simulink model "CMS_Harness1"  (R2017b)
settings: Solver=FixedStepDiscrete  StartTime=0.0  StopTime=2  FixedStep=0.01  RelTol=1e-3  EnableMultiTasking=on
undefined symbols (not defined in the file): sigbuilder_block
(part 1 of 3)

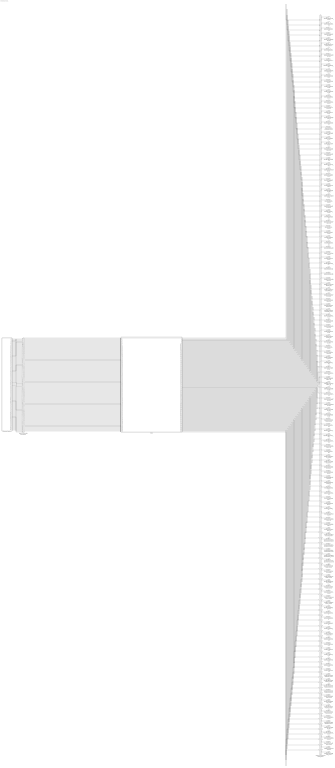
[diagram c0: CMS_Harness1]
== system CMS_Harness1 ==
  CMS : ModelReference  ModelNameDialog=CMS  SimulationMode=Normal  ModelReferenceVersion='M100C100'
  Harness Inputs : Subsystem  Tag=STV Subsys  LoadFcn=sigbuilder_block('load');  StartFcn=sigbuilder_block('start');  StopFcn=sigbuilder_block('stop');  ClipboardFcn=sigbuilder_block('clipboard');  mask(Sigbuilder block){tuvar=[0:10]}
      mask init:
      | if ~strcmp(get_param(bdroot(gcb),'SimulationStatus'),'stopped'),tuvar = sigbuilder_block('maskInit'); end
  Input Conversion Subsystem : Subsystem  Tag=__SLT_ICS__  Description=Signal spec. and routing
  Output Conversion Subsystem : Subsystem  Tag=__SLT_OCS__  Description=Signal spec. and routing
  GeCMS_HVConnSt_enum : Outport  OutDataTypeStr=uint8  PortDimensions=[1]
  GbCMS_NegCtlSt_flg : Outport  Port=2  OutDataTypeStr=boolean  PortDimensions=[1]
  GbCMS_PosCtlSt_flg : Outport  Port=3  OutDataTypeStr=boolean  PortDimensions=[1]
  GbCMS_ChrgPosCtlSt_flg : Outport  Port=4  OutDataTypeStr=boolean  PortDimensions=[1]
  GbCMS_ChrgNegCtlSt_flg : Outport  Port=5  OutDataTypeStr=boolean  PortDimensions=[1]
  GeCMS_RelStuckClosed_enum : Outport  Port=6  OutDataTypeStr=uint8  PortDimensions=[1]
  GcCMS_PackVolt_V : Outport  Port=7  OutDataTypeStr=fixdt('ufix16_Sp1')  PortDimensions=[1]
  GbCMS_PreChrgCtlSt_flg : Outport  Port=8  OutDataTypeStr=boolean  PortDimensions=[1]
  GcCMS_BattCurr_A : Outport  Port=9  OutDataTypeStr=fixdt('ufix16_Sp1_Bn700')  PortDimensions=[1]
  GbCMS_Kl15WkUp_flg : Outport  Port=10  OutDataTypeStr=boolean  PortDimensions=[1]
  GbCMS_ThmRunAway_flg : Outport  Port=11  OutDataTypeStr=boolean  PortDimensions=[1]
  GcCMS_CoolTempIn_C : Outport  Port=12  OutDataTypeStr=fixdt('ufix8_Bn40')  PortDimensions=[1]
  GcCMS_CoolTempOut_C : Outport  Port=13  OutDataTypeStr=fixdt('ufix8_Bn40')  PortDimensions=[1]
  GcCMS_CoolPwrReq_W : Outport  Port=14  OutDataTypeStr=fixdt('ufix16_Sp1')  PortDimensions=[1]
  GcCMS_HeatPwrReq_W : Outport  Port=15  OutDataTypeStr=fixdt('ufix16_Sp1')  PortDimensions=[1]
  GeCMS_CoolReq_enum : Outport  Port=16  OutDataTypeStr=uint8  PortDimensions=[1]
  GeCMS_HeatReq_enum : Outport  Port=17  OutDataTypeStr=uint8  PortDimensions=[1]
  GcCMS_PeakCurrDisCh_A : Outport  Port=18  OutDataTypeStr=fixdt('ufix16_Sp1')  PortDimensions=[1]
  GcCMS_PeakCurrCh_A : Outport  Port=19  OutDataTypeStr=fixdt('ufix16_Sp1_Bn1500')  PortDimensions=[1]
  GcCMS_PeakVoltDisCh_V : Outport  Port=20  OutDataTypeStr=uint16  PortDimensions=[1]
  GcCMS_PeakVoltCh_V : Outport  Port=21  OutDataTypeStr=uint16  PortDimensions=[1]
  GeCMS_Thm_propagat_enum : Outport  Port=22  OutDataTypeStr=uint8  PortDimensions=[1]
  GcCMS_ClntTgtTemp_C : Outport  Port=23  OutDataTypeStr=fixdt('ufix8_Bn40')  PortDimensions=[1]
  GcCMS_HtTgtTemp_C : Outport  Port=24  OutDataTypeStr=fixdt('ufix8_Bn40')  PortDimensions=[1]
  GcCMS_MaxCellVolt_V : Outport  Port=25  OutDataTypeStr=fixdt('ufix16_Sp001')  PortDimensions=[1]
  GcCMS_BusbarTempMax_C : Outport  Port=26  OutDataTypeStr=fixdt('ufix8_Bn40')  PortDimensions=[1]
  GcCMS_BusbarTempMin_C : Outport  Port=27  OutDataTypeStr=fixdt('ufix8_Bn40')  PortDimensions=[1]
  GcCMS_MinCellVolt_V : Outport  Port=28  OutDataTypeStr=fixdt('ufix16_Sp001')  PortDimensions=[1]
  GbCMS_ChrgCmd_flg : Outport  Port=29  OutDataTypeStr=boolean  PortDimensions=[1]
  GcCMS_ActPwrChrg_Kw : Outport  Port=30  OutDataTypeStr=fixdt('ufix16_Sp1')  PortDimensions=[1]
  GcCMS_MaxVoltChrg_V : Outport  Port=31  OutDataTypeStr=fixdt('ufix16_Sp1')  PortDimensions=[1]
  GcCMS_ReqVoltChrg_V : Outport  Port=32  OutDataTypeStr=fixdt('ufix16_Sp1')  PortDimensions=[1]
  GcCMS_ReqCurrChrg_A : Outport  Port=33  OutDataTypeStr=fixdt('ufix16_Sp1_Bn700')  PortDimensions=[1]
  GbCMS_ObcRdyReq_flg : Outport  Port=34  OutDataTypeStr=boolean  PortDimensions=[1]
  GbCMS_DischgCmd_flg : Outport  Port=35  OutDataTypeStr=boolean  PortDimensions=[1]
  GeCMS_BmsSt_enum : Outport  Port=36  OutDataTypeStr=uint8  PortDimensions=[1]
  GeCMS_BmsSelfChk_enum : Outport  Port=37  OutDataTypeStr=uint8  PortDimensions=[1]
  GeCMS_IsoFault_enum : Outport  Port=38  OutDataTypeStr=uint8  PortDimensions=[1]
  GcCMS_SocDspl_pct : Outport  Port=39  OutDataTypeStr=uint8  PortDimensions=[1]
  GbCMS_HvilOpenFault_flg : Outport  Port=40  OutDataTypeStr=boolean  PortDimensions=[1]
  GeCMS_FltLvl_enum : Outport  Port=41  OutDataTypeStr=uint8  PortDimensions=[1]
  GeCMS_V2xMod_enum : Outport  Port=42  OutDataTypeStr=uint8  PortDimensions=[1]
  GcCMS_ChgSOCset_pct : Outport  Port=43  OutDataTypeStr=fixdt('ufix8_B80')  PortDimensions=[1]
  GcCMS_BattSoh_pct : Outport  Port=44  OutDataTypeStr=uint8  PortDimensions=[1]
  GcCMS_SOCA_pct : Outport  Port=45  OutDataTypeStr=uint8  PortDimensions=[1]
  GeCMS_IviDischg_enum : Outport  Port=46  OutDataTypeStr=uint8  PortDimensions=[1]
  GcCMS_PackCurLem_A : Outport  Port=47  OutDataTypeStr=fixdt('ufix16_Bn1023')  PortDimensions=[1]
  GcCMS_BattInVolt_V : Outport  Port=48  OutDataTypeStr=fixdt('ufix16_Sp1')  PortDimensions=[1]
  GbCMS_BalSt_flg : Outport  Port=49  OutDataTypeStr=boolean  PortDimensions=[1]
  GbCMS_BalVlg_flg : Outport  Port=50  OutDataTypeStr=boolean  PortDimensions=[1]
  GbCMS_VcuPwrUpReq_flg : Outport  Port=51  OutDataTypeStr=boolean  PortDimensions=[1]
  GbCMS_VcuPwrUpReqVld_flg : Outport  Port=52  OutDataTypeStr=boolean  PortDimensions=[1]
  GcCMS_ConstCurrDisChMax_A : Outport  Port=53  OutDataTypeStr=fixdt('ufix16_Sp1')  PortDimensions=[1]
  GcCMS_ConstCurrChMax_A : Outport  Port=54  OutDataTypeStr=fixdt('ufix16_Sp1_Bn700')  PortDimensions=[1]
  GbCMS_PwrDownReq_flg : Outport  Port=55  OutDataTypeStr=boolean  PortDimensions=[1]
  GbCMS_PwrDownReqVld_flg : Outport  Port=56  OutDataTypeStr=boolean  PortDimensions=[1]
  GeCMS_ChrgPreThmMode_enum : Outport  Port=57  OutDataTypeStr=uint8  PortDimensions=[1]
  GeCMS_ElockReq_enum : Outport  Port=58  OutDataTypeStr=uint8  PortDimensions=[1]
  GeCMS_PreThmReq_enum : Outport  Port=59  OutDataTypeStr=uint8  PortDimensions=[1]
  GcCMS_PeakPwrDisCh_Kw : Outport  Port=60  OutDataTypeStr=fixdt('ufix16_Sp1')  PortDimensions=[1]
  GcCMS_PeakPwrCh_Kw : Outport  Port=61  OutDataTypeStr=fixdt('ufix16_Sp1')  PortDimensions=[1]
  GcCMS_ConstPwrDisCh_Kw : Outport  Port=62  OutDataTypeStr=fixdt('ufix16_Sp1')  PortDimensions=[1]
  GcCMS_ConstPwrCh_Kw : Outport  Port=63  OutDataTypeStr=fixdt('ufix16_Sp1')  PortDimensions=[1]
  GcCMS_ResIso_Kohm : Outport  Port=64  OutDataTypeStr=uint16  PortDimensions=[1]
  GcCMS_ChrgRemTime_Min : Outport  Port=65  OutDataTypeStr=uint16  PortDimensions=[1]
  GeCMS_ACPlugCnnt_enum : Outport  Port=66  OutDataTypeStr=uint8  PortDimensions=[1]
  GbCMS_BattFull_flg : Outport  Port=67  OutDataTypeStr=boolean  PortDimensions=[1]
  GbCMS_WarnLamp_flg : Outport  Port=68  OutDataTypeStr=boolean  PortDimensions=[1]
  GbCMS_SerLamp_flg : Outport  Port=69  OutDataTypeStr=boolean  PortDimensions=[1]
  GbCMS_TempDiffWarn_flg : Outport  Port=70  OutDataTypeStr=boolean  PortDimensions=[1]
  GbCMS_OverChrgWarn_flg : Outport  Port=71  OutDataTypeStr=boolean  PortDimensions=[1]
  GbCMS_ConsisWarn_flg : Outport  Port=72  OutDataTypeStr=boolean  PortDimensions=[1]
  GbCMS_MishWarn_flg : Outport  Port=73  OutDataTypeStr=boolean  PortDimensions=[1]
  GbCMS_SocHopWarn_flg : Outport  Port=74  OutDataTypeStr=boolean  PortDimensions=[1]
  GbCMS_SocHighWarn_flg : Outport  Port=75  OutDataTypeStr=boolean  PortDimensions=[1]
  GbCMS_SocLowWarn_flg : Outport  Port=76  OutDataTypeStr=boolean  PortDimensions=[1]
  GbCMS_OTAModeSt_flg : Outport  Port=77  OutDataTypeStr=boolean  PortDimensions=[1]
  GeCMS_AcDcConnBoth_enum : Outport  Port=78  OutDataTypeStr=uint8  PortDimensions=[1]
  GbCMS_CellUvFlt_flg : Outport  Port=79  OutDataTypeStr=boolean  PortDimensions=[1]
  GbCMS_CellOvFlt_flg : Outport  Port=80  OutDataTypeStr=boolean  PortDimensions=[1]
  GbCMS_PackUvFlt_flg : Outport  Port=81  OutDataTypeStr=boolean  PortDimensions=[1]
  GbCMS_PackOvFlt_flg : Outport  Port=82  OutDataTypeStr=boolean  PortDimensions=[1]
  GbCMS_TempHighWarn_flg : Outport  Port=83  OutDataTypeStr=boolean  PortDimensions=[1]
  GcCMS_RealSoc_pct : Outport  Port=84  OutDataTypeStr=uint8  PortDimensions=[1]
  GeCMS_DCPlugConn_enum : Outport  Port=85  OutDataTypeStr=uint8  PortDimensions=[1]
  GeCMS_ACChgMode_enum : Outport  Port=86  OutDataTypeStr=uint8  PortDimensions=[1]
  GeCMS_DCChgMode_enum : Outport  Port=87  OutDataTypeStr=uint8  PortDimensions=[1]
  GcCMS_BattTempAvrg_C : Outport  Port=88  OutDataTypeStr=fixdt('ufix8_Bn40')  PortDimensions=[1]
  GcCMS_BattNrmEnrg_kwh : Outport  Port=89  OutDataTypeStr=fixdt('ufix16_Sp01')  PortDimensions=[1]
  GbCMS_BattTempFault_flg : Outport  Port=90  OutDataTypeStr=boolean  PortDimensions=[1]
  GcCMS_BattSoe_kwh : Outport  Port=91  OutDataTypeStr=fixdt('ufix16_Sp1')  PortDimensions=[1]
  GbCMS_IsoChkSt_flg : Outport  Port=92  OutDataTypeStr=boolean  PortDimensions=[1]
  GcCMS_BattTempMax_C : Outport  Port=93  OutDataTypeStr=fixdt('ufix8_Bn40')  PortDimensions=[1]
  GcCMS_BattTempMin_C : Outport  Port=94  OutDataTypeStr=fixdt('ufix8_Bn40')  PortDimensions=[1]
  GcCMS_FuseVolt_V : Outport  Port=95  OutDataTypeStr=fixdt('ufix8_E1')  PortDimensions=[1]
  GcCMS_ChrgAccum_Ah : Outport  Port=96  OutDataTypeStr=uint8  PortDimensions=[1]
  GbCMS_DChgStVoltOut_flg : Outport  Port=97  OutDataTypeStr=boolean  PortDimensions=[1]
  GcCMS_DChrgVoltReq_V : Outport  Port=98  OutDataTypeStr=fixdt('ufix16_Sp1')  PortDimensions=[1]
  GcCMS_DChrgCurrReq_A : Outport  Port=99  OutDataTypeStr=fixdt('ufix16_Sp1_Bn400')  PortDimensions=[1]
  GcCMS_DChrgRchSocLmt_numb : Outport  Port=100  OutDataTypeStr=uint8  PortDimensions=[1]
  GcCMS_DChrgRchPackVoltLmt_numb : Outport  Port=101  OutDataTypeStr=uint8  PortDimensions=[1]
  GcCMS_DChrgRchCellVoltLmt_numb : Outport  Port=102  OutDataTypeStr=uint8  PortDimensions=[1]
  GcCMS_DChrgChrgerActStop_numb : Outport  Port=103  OutDataTypeStr=uint8  PortDimensions=[1]
  GcCMS_DChrgBattInsulationErr_numb : Outport  Port=104  OutDataTypeStr=uint8  PortDimensions=[1]
  GcCMS_DChrgOutpCnntOvrTempErr_numb : Outport  Port=105  OutDataTypeStr=uint8  PortDimensions=[1]
  GcCMS_PcbOvrTempErr_numb : Outport  Port=106  OutDataTypeStr=uint8  PortDimensions=[1]
  GcCMS_ChrgCnntErr_numb : Outport  Port=107  OutDataTypeStr=uint8  PortDimensions=[1]
  GcCMS_BattOvrTempErr_numb : Outport  Port=108  OutDataTypeStr=uint8  PortDimensions=[1]
  GcCMS_MainRelayErr_numb : Outport  Port=109  OutDataTypeStr=uint8  PortDimensions=[1]
  GcCMS_CC2ChkVoltErr_numb : Outport  Port=110  OutDataTypeStr=uint8  PortDimensions=[1]
  GcCMS_OtherErr_numb : Outport  Port=111  OutDataTypeStr=uint8  PortDimensions=[1]
  GcCMS_ChrgCurrAbnrm_numb : Outport  Port=112  OutDataTypeStr=uint8  PortDimensions=[1]
  GcCMS_ChrgVoltAbnrm_numb : Outport  Port=113  OutDataTypeStr=uint8  PortDimensions=[1]
  GcCMS_CellVoltCnt_numb : Outport  Port=114  OutDataTypeStr=uint8  PortDimensions=[1]
  GcCMS_CellVolt1_V : Outport  Port=115  OutDataTypeStr=fixdt('ufix16_Sp001')  PortDimensions=[1]
  GcCMS_CellVolt2_V : Outport  Port=116  OutDataTypeStr=fixdt('ufix16_Sp001')  PortDimensions=[1]
  GcCMS_CellVolt3_V : Outport  Port=117  OutDataTypeStr=fixdt('ufix16_Sp001')  PortDimensions=[1]
  GcCMS_CellVolt4_V : Outport  Port=118  OutDataTypeStr=fixdt('ufix16_Sp001')  PortDimensions=[1]
  GcCMS_CellTempCnt_numb : Outport  Port=119  OutDataTypeStr=uint8  PortDimensions=[1]
  GcCMS_CellTemp1_C : Outport  Port=120  OutDataTypeStr=fixdt('ufix8_Bn40')  PortDimensions=[1]
  GcCMS_CellTemp2_C : Outport  Port=121  OutDataTypeStr=fixdt('ufix8_Bn40')  PortDimensions=[1]
  GcCMS_CellTemp3_C : Outport  Port=122  OutDataTypeStr=fixdt('ufix8_Bn40')  PortDimensions=[1]
  GcCMS_CellTemp4_C : Outport  Port=123  OutDataTypeStr=fixdt('ufix8_Bn40')  PortDimensions=[1]
  GcCMS_CellTemp5_C : Outport  Port=124  OutDataTypeStr=fixdt('ufix8_Bn40')  PortDimensions=[1]
  GcCMS_CellTemp6_C : Outport  Port=125  OutDataTypeStr=fixdt('ufix8_Bn40')  PortDimensions=[1]
  GcCMS_CellTemp7_C : Outport  Port=126  OutDataTypeStr=fixdt('ufix8_Bn40')  PortDimensions=[1]
  GcCMS_MaxCellVoltNumb_numb : Outport  Port=127  OutDataTypeStr=uint8  PortDimensions=[1]
  GcCMS_MinCellVoltNumb_numb : Outport  Port=128  OutDataTypeStr=uint8  PortDimensions=[1]
  GcCMS_MaxCellTempNumb_numb : Outport  Port=129  OutDataTypeStr=uint8  PortDimensions=[1]
  GcCMS_MinCellTempNumb_numb : Outport  Port=130  OutDataTypeStr=uint8  PortDimensions=[1]
  GcCMS_MaxVoltNumb_numb : Outport  Port=131  OutDataTypeStr=uint8  PortDimensions=[1]
  GcCMS_MinVoltNumb_numb : Outport  Port=132  OutDataTypeStr=uint8  PortDimensions=[1]
  GcCMS_MaxTempNumb_numb : Outport  Port=133  OutDataTypeStr=uint8  PortDimensions=[1]
  GcCMS_MinTempNumb_numb : Outport  Port=134  OutDataTypeStr=uint8  PortDimensions=[1]
  GeCMS_ChgMode_enum : Outport  Port=135  OutDataTypeStr=uint8  PortDimensions=[1]
  GeCMS_DChrgModeDebug_enum : Outport  Port=136  OutDataTypeStr=uint8  PortDimensions=[1]
  GbCMS_DChrgWkUp_flg : Outport  Port=137  OutDataTypeStr=boolean  PortDimensions=[1]
  GeCMS_EvccMode_enum : Outport  Port=138  OutDataTypeStr=uint8  PortDimensions=[1]
  GeCMS_AChrgObsr_enum : Outport  Port=139  OutDataTypeStr=uint8  PortDimensions=[1]
  GeCMS_PreThmObsvr_enum : Outport  Port=140  OutDataTypeStr=uint8  PortDimensions=[1]
  GbCMS_StartCanSend_flg : Outport  Port=141  OutDataTypeStr=boolean  PortDimensions=[1]
  GeCMS_AppChgMode_enum : Outport  Port=142  OutDataTypeStr=uint8  PortDimensions=[1]
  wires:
  Harness Inputs/1(GeCTC_CtrCtlState_enum) -> Input Conversion Subsystem/1(Inport_1)
  Harness Inputs/2(GbCTC_NegCtlState_flg) -> Input Conversion Subsystem/2(Inport_2)
  Harness Inputs/3(GbCTC_PosCtlState_flg) -> Input Conversion Subsystem/3(Inport_3)
  Harness Inputs/4(GbCTC_DCPosChrgCtlState_flg) -> Input Conversion Subsystem/4(Inport_4)
  Harness Inputs/5(GbCTC_DCNegChrgCtlState_flg) -> Input Conversion Subsystem/5(Inport_5)
  Harness Inputs/6(GcHDP_PackVolt_V) -> Input Conversion Subsystem/6(Inport_6)
  Harness Inputs/7(GbCTC_PreChrgCtlState_flg) -> Input Conversion Subsystem/7(Inport_7)
  Harness Inputs/8(GcHDP_PackCrnt_A) -> Input Conversion Subsystem/8(Inport_8)
  Harness Inputs/9(GbWSM_Kl15WkUpPrs_flg) -> Input Conversion Subsystem/9(Inport_9)
  Harness Inputs/10(GcCDP_MinCellVolt_mV) -> Input Conversion Subsystem/10(Inport_10)
  Harness Inputs/11(GcCDP_MaxCellVolt_mV) -> Input Conversion Subsystem/11(Inport_11)
  Harness Inputs/12(GbACC_ObcChrgCmd_flg) -> Input Conversion Subsystem/12(Inport_12)
  Harness Inputs/13(GcACC_ACChrgVoltRqst_V) -> Input Conversion Subsystem/13(Inport_13)
  Harness Inputs/14(GcACC_ACChrgCrntRqst_A) -> Input Conversion Subsystem/14(Inport_14)
  Harness Inputs/15(GbACC_ACChrgRqst_flg) -> Input Conversion Subsystem/15(Inport_15)
  Harness Inputs/16(GeCTC_CtrCtlConnMode_enum) -> Input Conversion Subsystem/16(Inport_16)
  Harness Inputs/17(GbMSM_SelfCheck_flg) -> Input Conversion Subsystem/17(Inport_17)
  Harness Inputs/18(GcSOC_DispSOC_pct) -> Input Conversion Subsystem/18(Inport_18)
  Harness Inputs/19(GbISP_TFHvilLFlt_flg) -> Input Conversion Subsystem/19(Inport_19)
  Harness Inputs/20(GbFTC_OpenContactor_flg) -> Input Conversion Subsystem/20(Inport_20)
  Harness Inputs/21(GcSOH_PackSOH_pct) -> Input Conversion Subsystem/21(Inport_21)
  Harness Inputs/22(GcSOC_PackSOC_pct) -> Input Conversion Subsystem/22(Inport_22)
  Harness Inputs/23(GcHDP_HallCrnt_A) -> Input Conversion Subsystem/23(Inport_23)
  Harness Inputs/24(GbMSM_SelfChckMaxTiReach_flg) -> Input Conversion Subsystem/24(Inport_24)
  Harness Inputs/25(GbDCC_DCChrgRqst_flg) -> Input Conversion Subsystem/25(Inport_25)
  Harness Inputs/26(GcSOP_DischrgConstPwr_kW) -> Input Conversion Subsystem/26(Inport_26)
  Harness Inputs/27(GcSOP_ChrgConstPwr_kW) -> Input Conversion Subsystem/27(Inport_27)
  Harness Inputs/28(GcISO_HVIsoValue_kohm) -> Input Conversion Subsystem/28(Inport_28)
  Harness Inputs/29(GeODP_ObcCcSt_enum) -> Input Conversion Subsystem/29(Inport_29)
  Harness Inputs/30(GbDCC_DCChrgFinish_flg) -> Input Conversion Subsystem/30(Inport_30)
  Harness Inputs/31(GbACC_ACChrgFinish_flg) -> Input Conversion Subsystem/31(Inport_31)
  Harness Inputs/32(GeACC_ACChrgState_enum) -> Input Conversion Subsystem/32(Inport_32)
  Harness Inputs/33(GeDCC_DCConnSt_enum) -> Input Conversion Subsystem/33(Inport_33)
  Harness Inputs/34(GeLDP_CC2St_enum) -> Input Conversion Subsystem/34(Inport_34)
  Harness Inputs/35(GcCDP_AvgCellTemp_C) -> Input Conversion Subsystem/35(Inport_35)
  Harness Inputs/36(GbISO_IsoForbid_flg) -> Input Conversion Subsystem/36(Inport_36)
  Harness Inputs/37(GcCDP_MaxCellTemp_C) -> Input Conversion Subsystem/37(Inport_37)
  Harness Inputs/38(GcCDP_MinCellTemp_C) -> Input Conversion Subsystem/38(Inport_38)
  Harness Inputs/39(GcDCS_3072ChrgVoltReq_V) -> Input Conversion Subsystem/39(Inport_39)
  Harness Inputs/40(GcDCC_DCChrgCrntRqst_A) -> Input Conversion Subsystem/40(Inport_40)
  Harness Inputs/41(GcLDP_lntWtTemp_C) -> Input Conversion Subsystem/41(Inport_41)
  Harness Inputs/42(GcLDP_OutWtTemp_C) -> Input Conversion Subsystem/42(Inport_42)
  Harness Inputs/43(GcBTM_CoolPwrReq_W) -> Input Conversion Subsystem/43(Inport_43)
  Harness Inputs/44(GcBTM_HeatPwrReq_W) -> Input Conversion Subsystem/44(Inport_44)
  Harness Inputs/45(GeBTM_CoolReq_enum) -> Input Conversion Subsystem/45(Inport_45)
  Harness Inputs/46(GeBTM_HeatReq_enum) -> Input Conversion Subsystem/46(Inport_46)
  Harness Inputs/47(GbODP_V2XDischrgCmd_flg) -> Input Conversion Subsystem/47(Inport_47)
  Harness Inputs/48(GeMSM_BMUState_enum) -> Input Conversion Subsystem/48(Inport_48)
  Harness Inputs/49(GcHDP_FuseVolt_V) -> Input Conversion Subsystem/49(Inport_49)
  Harness Inputs/50(GbADP_DischgReq_flg) -> Input Conversion Subsystem/50(Inport_50)
  Harness Inputs/51(GcHDP_PosCtlVolt_V) -> Input Conversion Subsystem/51(Inport_51)
  Harness Inputs/52(GcCDP_MaxCellVoltNumb_numb) -> Input Conversion Subsystem/52(Inport_52)
  Harness Inputs/53(GcCDP_MinCellVoltNumb_numb) -> Input Conversion Subsystem/53(Inport_53)
  Harness Inputs/54(GcCDP_MaxCellTempNumb_numb) -> Input Conversion Subsystem/54(Inport_54)
  Harness Inputs/55(GcCDP_MinCellTempNumb_numb) -> Input Conversion Subsystem/55(Inport_55)
  Harness Inputs/56(GbWSM_DCWkUpPrs_flg) -> Input Conversion Subsystem/56(Inport_56)
  Harness Inputs/57(GbACC_PreThmObcChrgCmd_flg) -> Input Conversion Subsystem/57(Inport_57)
  Harness Inputs/58(GbACC_PreThmRqst_flg) -> Input Conversion Subsystem/58(Inport_58)
  Harness Inputs/59(GcACC_PreThmCrntRqst_A) -> Input Conversion Subsystem/59(Inport_59)
  Harness Inputs/60(GcACC_PreThmVoltRqst_V) -> Input Conversion Subsystem/60(Inport_60)
  Harness Inputs/61(GbACC_PreHeatPrmt_flg) -> Input Conversion Subsystem/61(Inport_61)
  Harness Inputs/62(GbFTC_PowerDown_flg) -> Input Conversion Subsystem/62(Inport_62)
  Harness Inputs/63(GcBTM_CoolTempReq_C) -> Input Conversion Subsystem/63(Inport_63)
  Harness Inputs/64(GcBTM_HeatTempReq_C) -> Input Conversion Subsystem/64(Inport_64)
  Harness Inputs/65(GcACC_ChrgingTiRem_min) -> Input Conversion Subsystem/65(Inport_65)
  Harness Inputs/66(GcDCC_ChrgingTiRem_min) -> Input Conversion Subsystem/66(Inport_66)
  Harness Inputs/67(GeVDP_PreThmEna_enum) -> Input Conversion Subsystem/67(Inport_67)
  Harness Inputs/68(GcSOP_DischrgPwr_kW) -> Input Conversion Subsystem/68(Inport_68)
  Harness Inputs/69(GcSOP_ChrgPwr_kW) -> Input Conversion Subsystem/69(Inport_69)
  Harness Inputs/70(GbFTC_DischrgPwrLimitLevel3_flg) -> Input Conversion Subsystem/70(Inport_70)
  Harness Inputs/71(GbFTC_RegenPwrLimitLevel3_flg) -> Input Conversion Subsystem/71(Inport_71)
  Harness Inputs/72(GbFTC_DischrgPwrLimitLevel2_flg) -> Input Conversion Subsystem/72(Inport_72)
  Harness Inputs/73(GbFTC_RegenPwrLimitLevel2_flg) -> Input Conversion Subsystem/73(Inport_73)
  Harness Inputs/74(GbFTC_DCChrgCurrLimitLevel2_flg) -> Input Conversion Subsystem/74(Inport_74)
  Harness Inputs/75(GbFTC_ACChrgCurrLimitLevel2_flg) -> Input Conversion Subsystem/75(Inport_75)
  Harness Inputs/76(GbFTC_DischrgPwrLimitLevel1_flg) -> Input Conversion Subsystem/76(Inport_76)
  Harness Inputs/77(GbFTC_RegenPwrLimitLevel1_flg) -> Input Conversion Subsystem/77(Inport_77)
  Harness Inputs/78(GcCDP_MaxBusbarTemp_C) -> Input Conversion Subsystem/78(Inport_78)
  Harness Inputs/79(GcCDP_MinBusbarTemp_C) -> Input Conversion Subsystem/79(Inport_79)
  Harness Inputs/80(GeDCC_DCChrgState_enum) -> Input Conversion Subsystem/80(Inport_80)
  Harness Inputs/81(GeLDP_ChrgGunConnSt_enum) -> Input Conversion Subsystem/81(Inport_81)
  Harness Inputs/82(GbISP_TFThmRnwyfDet_flg) -> Input Conversion Subsystem/82(Inport_82)
  Harness Inputs/83(GcUDS_CellTempNumb_numb) -> Input Conversion Subsystem/83(Inport_83)
  Harness Inputs/84(GcUDS_BusbarTempNumb_numb) -> Input Conversion Subsystem/84(Inport_84)
  Harness Inputs/85(GcUDS_CellVoltNum_numb) -> Input Conversion Subsystem/85(Inport_85)
  Harness Inputs/86(GcUDS_BatEnergy_kWh) -> Input Conversion Subsystem/86(Inport_86)
  Harness Inputs/87(GbACC_HoldTempPrmt_flg) -> Input Conversion Subsystem/87(Inport_87)
  Harness Inputs/88(GbACC_HoldTempObcChrgCmd_flg) -> Input Conversion Subsystem/88(Inport_88)
  Harness Inputs/89(GcACC_HoldTempVoltRqst_V) -> Input Conversion Subsystem/89(Inport_89)
  Harness Inputs/90(GcACC_HoldTempCrntRqst_A) -> Input Conversion Subsystem/90(Inport_90)
  Harness Inputs/91(GbACC_HoldTempRqst_flg) -> Input Conversion Subsystem/91(Inport_91)
  Harness Inputs/92(GbISP_TFIsoResFltLevel2_flg) -> Input Conversion Subsystem/92(Inport_92)
  Harness Inputs/93(GbISP_TFIsoDCResFltLevel2_flg) -> Input Conversion Subsystem/93(Inport_93)
  Harness Inputs/94(GbISP_TFIsoHVoffResFltLevel2_flg) -> Input Conversion Subsystem/94(Inport_94)
  Harness Inputs/95(GbISP_TFIsoResFltLevel1_flg) -> Input Conversion Subsystem/95(Inport_95)
  Harness Inputs/96(GbISP_TFIsoDCResFltLevel1_flg) -> Input Conversion Subsystem/96(Inport_96)
  Harness Inputs/97(GbISP_TFIsoHVoffResFltLevel1_flg) -> Input Conversion Subsystem/97(Inport_97)
  Harness Inputs/98(GbFTC_Level1FltReaction_flg) -> Input Conversion Subsystem/98(Inport_98)
  Output Conversion Subsystem/1(Outport_1) -> GeCMS_HVConnSt_enum/1
  Output Conversion Subsystem/2(Outport_2) -> GbCMS_NegCtlSt_flg/1
  Output Conversion Subsystem/3(Outport_3) -> GbCMS_PosCtlSt_flg/1
  Output Conversion Subsystem/4(Outport_4) -> GbCMS_ChrgPosCtlSt_flg/1
  Output Conversion Subsystem/5(Outport_5) -> GbCMS_ChrgNegCtlSt_flg/1
  Output Conversion Subsystem/6(Outport_6) -> GeCMS_RelStuckClosed_enum/1
  Output Conversion Subsystem/7(Outport_7) -> GcCMS_PackVolt_V/1
  Output Conversion Subsystem/8(Outport_8) -> GbCMS_PreChrgCtlSt_flg/1
  Output Conversion Subsystem/9(Outport_9) -> GcCMS_BattCurr_A/1
  Output Conversion Subsystem/10(Outport_10) -> GbCMS_Kl15WkUp_flg/1
  Output Conversion Subsystem/11(Outport_11) -> GbCMS_ThmRunAway_flg/1
  Output Conversion Subsystem/12(Outport_12) -> GcCMS_CoolTempIn_C/1
  Output Conversion Subsystem/13(Outport_13) -> GcCMS_CoolTempOut_C/1
  Output Conversion Subsystem/14(Outport_14) -> GcCMS_CoolPwrReq_W/1
  Output Conversion Subsystem/15(Outport_15) -> GcCMS_HeatPwrReq_W/1
  Output Conversion Subsystem/16(Outport_16) -> GeCMS_CoolReq_enum/1
  Output Conversion Subsystem/17(Outport_17) -> GeCMS_HeatReq_enum/1
  Output Conversion Subsystem/18(Outport_18) -> GcCMS_PeakCurrDisCh_A/1
  Output Conversion Subsystem/19(Outport_19) -> GcCMS_PeakCurrCh_A/1
  Output Conversion Subsystem/20(Outport_20) -> GcCMS_PeakVoltDisCh_V/1
  Output Conversion Subsystem/21(Outport_21) -> GcCMS_PeakVoltCh_V/1
  Output Conversion Subsystem/22(Outport_22) -> GeCMS_Thm_propagat_enum/1
  Output Conversion Subsystem/23(Outport_23) -> GcCMS_ClntTgtTemp_C/1
  Output Conversion Subsystem/24(Outport_24) -> GcCMS_HtTgtTemp_C/1
  Output Conversion Subsystem/25(Outport_25) -> GcCMS_MaxCellVolt_V/1
  Output Conversion Subsystem/26(Outport_26) -> GcCMS_BusbarTempMax_C/1
  Output Conversion Subsystem/27(Outport_27) -> GcCMS_BusbarTempMin_C/1
  Output Conversion Subsystem/28(Outport_28) -> GcCMS_MinCellVolt_V/1
  Output Conversion Subsystem/29(Outport_29) -> GbCMS_ChrgCmd_flg/1
  Output Conversion Subsystem/30(Outport_30) -> GcCMS_ActPwrChrg_Kw/1
  Output Conversion Subsystem/31(Outport_31) -> GcCMS_MaxVoltChrg_V/1
  Output Conversion Subsystem/32(Outport_32) -> GcCMS_ReqVoltChrg_V/1
  Output Conversion Subsystem/33(Outport_33) -> GcCMS_ReqCurrChrg_A/1
  Output Conversion Subsystem/34(Outport_34) -> GbCMS_ObcRdyReq_flg/1
  Output Conversion Subsystem/35(Outport_35) -> GbCMS_DischgCmd_flg/1
  Output Conversion Subsystem/36(Outport_36) -> GeCMS_BmsSt_enum/1
  Output Conversion Subsystem/37(Outport_37) -> GeCMS_BmsSelfChk_enum/1
  Output Conversion Subsystem/38(Outport_38) -> GeCMS_IsoFault_enum/1
  Output Conversion Subsystem/39(Outport_39) -> GcCMS_SocDspl_pct/1
  Output Conversion Subsystem/40(Outport_40) -> GbCMS_HvilOpenFault_flg/1
  Output Conversion Subsystem/41(Outport_41) -> GeCMS_FltLvl_enum/1
  Output Conversion Subsystem/42(Outport_42) -> GeCMS_V2xMod_enum/1
  Output Conversion Subsystem/43(Outport_43) -> GcCMS_ChgSOCset_pct/1
  Output Conversion Subsystem/44(Outport_44) -> GcCMS_BattSoh_pct/1
  Output Conversion Subsystem/45(Outport_45) -> GcCMS_SOCA_pct/1
  Output Conversion Subsystem/46(Outport_46) -> GeCMS_IviDischg_enum/1
  Output Conversion Subsystem/47(Outport_47) -> GcCMS_PackCurLem_A/1
  Output Conversion Subsystem/48(Outport_48) -> GcCMS_BattInVolt_V/1
  Output Conversion Subsystem/49(Outport_49) -> GbCMS_BalSt_flg/1
  Output Conversion Subsystem/50(Outport_50) -> GbCMS_BalVlg_flg/1
  Output Conversion Subsystem/51(Outport_51) -> GbCMS_VcuPwrUpReq_flg/1
  Output Conversion Subsystem/52(Outport_52) -> GbCMS_VcuPwrUpReqVld_flg/1
  Output Conversion Subsystem/53(Outport_53) -> GcCMS_ConstCurrDisChMax_A/1
  Output Conversion Subsystem/54(Outport_54) -> GcCMS_ConstCurrChMax_A/1
  Output Conversion Subsystem/55(Outport_55) -> GbCMS_PwrDownReq_flg/1
  Output Conversion Subsystem/56(Outport_56) -> GbCMS_PwrDownReqVld_flg/1
  Output Conversion Subsystem/57(Outport_57) -> GeCMS_ChrgPreThmMode_enum/1
  Output Conversion Subsystem/58(Outport_58) -> GeCMS_ElockReq_enum/1
  Output Conversion Subsystem/59(Outport_59) -> GeCMS_PreThmReq_enum/1
  Output Conversion Subsystem/60(Outport_60) -> GcCMS_PeakPwrDisCh_Kw/1
  Output Conversion Subsystem/61(Outport_61) -> GcCMS_PeakPwrCh_Kw/1
  Output Conversion Subsystem/62(Outport_62) -> GcCMS_ConstPwrDisCh_Kw/1
  Output Conversion Subsystem/63(Outport_63) -> GcCMS_ConstPwrCh_Kw/1
  Output Conversion Subsystem/64(Outport_64) -> GcCMS_ResIso_Kohm/1
  Output Conversion Subsystem/65(Outport_65) -> GcCMS_ChrgRemTime_Min/1
  Output Conversion Subsystem/66(Outport_66) -> GeCMS_ACPlugCnnt_enum/1
  Output Conversion Subsystem/67(Outport_67) -> GbCMS_BattFull_flg/1
  Output Conversion Subsystem/68(Outport_68) -> GbCMS_WarnLamp_flg/1
  Output Conversion Subsystem/69(Outport_69) -> GbCMS_SerLamp_flg/1
  Output Conversion Subsystem/70(Outport_70) -> GbCMS_TempDiffWarn_flg/1
  Output Conversion Subsystem/71(Outport_71) -> GbCMS_OverChrgWarn_flg/1
  Output Conversion Subsystem/72(Outport_72) -> GbCMS_ConsisWarn_flg/1
  Output Conversion Subsystem/73(Outport_73) -> GbCMS_MishWarn_flg/1
  Output Conversion Subsystem/74(Outport_74) -> GbCMS_SocHopWarn_flg/1
  Output Conversion Subsystem/75(Outport_75) -> GbCMS_SocHighWarn_flg/1
  Output Conversion Subsystem/76(Outport_76) -> GbCMS_SocLowWarn_flg/1
  Output Conversion Subsystem/77(Outport_77) -> GbCMS_OTAModeSt_flg/1
  Output Conversion Subsystem/78(Outport_78) -> GeCMS_AcDcConnBoth_enum/1
  Output Conversion Subsystem/79(Outport_79) -> GbCMS_CellUvFlt_flg/1
  Output Conversion Subsystem/80(Outport_80) -> GbCMS_CellOvFlt_flg/1
  Output Conversion Subsystem/81(Outport_81) -> GbCMS_PackUvFlt_flg/1
  Output Conversion Subsystem/82(Outport_82) -> GbCMS_PackOvFlt_flg/1
  Output Conversion Subsystem/83(Outport_83) -> GbCMS_TempHighWarn_flg/1
  Output Conversion Subsystem/84(Outport_84) -> GcCMS_RealSoc_pct/1
  Output Conversion Subsystem/85(Outport_85) -> GeCMS_DCPlugConn_enum/1
  Output Conversion Subsystem/86(Outport_86) -> GeCMS_ACChgMode_enum/1
  Output Conversion Subsystem/87(Outport_87) -> GeCMS_DCChgMode_enum/1
  Output Conversion Subsystem/88(Outport_88) -> GcCMS_BattTempAvrg_C/1
  Output Conversion Subsystem/89(Outport_89) -> GcCMS_BattNrmEnrg_kwh/1
  Output Conversion Subsystem/90(Outport_90) -> GbCMS_BattTempFault_flg/1
  Output Conversion Subsystem/91(Outport_91) -> GcCMS_BattSoe_kwh/1
  Output Conversion Subsystem/92(Outport_92) -> GbCMS_IsoChkSt_flg/1
  Output Conversion Subsystem/93(Outport_93) -> GcCMS_BattTempMax_C/1
  Output Conversion Subsystem/94(Outport_94) -> GcCMS_BattTempMin_C/1
  Output Conversion Subsystem/95(Outport_95) -> GcCMS_FuseVolt_V/1
  Output Conversion Subsystem/96(Outport_96) -> GcCMS_ChrgAccum_Ah/1
  Output Conversion Subsystem/97(Outport_97) -> GbCMS_DChgStVoltOut_flg/1
  Output Conversion Subsystem/98(Outport_98) -> GcCMS_DChrgVoltReq_V/1
  Output Conversion Subsystem/99(Outport_99) -> GcCMS_DChrgCurrReq_A/1
  Output Conversion Subsystem/100(Outport_100) -> GcCMS_DChrgRchSocLmt_numb/1
  Output Conversion Subsystem/101(Outport_101) -> GcCMS_DChrgRchPackVoltLmt_numb/1
  Output Conversion Subsystem/102(Outport_102) -> GcCMS_DChrgRchCellVoltLmt_numb/1
  Output Conversion Subsystem/103(Outport_103) -> GcCMS_DChrgChrgerActStop_numb/1
  Output Conversion Subsystem/104(Outport_104) -> GcCMS_DChrgBattInsulationErr_numb/1
  Output Conversion Subsystem/105(Outport_105) -> GcCMS_DChrgOutpCnntOvrTempErr_numb/1
  Output Conversion Subsystem/106(Outport_106) -> GcCMS_PcbOvrTempErr_numb/1
  Output Conversion Subsystem/107(Outport_107) -> GcCMS_ChrgCnntErr_numb/1
  Output Conversion Subsystem/108(Outport_108) -> GcCMS_BattOvrTempErr_numb/1
  Output Conversion Subsystem/109(Outport_109) -> GcCMS_MainRelayErr_numb/1
  Output Conversion Subsystem/110(Outport_110) -> GcCMS_CC2ChkVoltErr_numb/1
  Output Conversion Subsystem/111(Outport_111) -> GcCMS_OtherErr_numb/1
  Output Conversion Subsystem/112(Outport_112) -> GcCMS_ChrgCurrAbnrm_numb/1
  Output Conversion Subsystem/113(Outport_113) -> GcCMS_ChrgVoltAbnrm_numb/1
  Output Conversion Subsystem/114(Outport_114) -> GcCMS_CellVoltCnt_numb/1
  Output Conversion Subsystem/115(Outport_115) -> GcCMS_CellVolt1_V/1
  Output Conversion Subsystem/116(Outport_116) -> GcCMS_CellVolt2_V/1
  Output Conversion Subsystem/117(Outport_117) -> GcCMS_CellVolt3_V/1
  Output Conversion Subsystem/118(Outport_118) -> GcCMS_CellVolt4_V/1
  Output Conversion Subsystem/119(Outport_119) -> GcCMS_CellTempCnt_numb/1
  Output Conversion Subsystem/120(Outport_120) -> GcCMS_CellTemp1_C/1
  Output Conversion Subsystem/121(Outport_121) -> GcCMS_CellTemp2_C/1
  Output Conversion Subsystem/122(Outport_122) -> GcCMS_CellTemp3_C/1
  Output Conversion Subsystem/123(Outport_123) -> GcCMS_CellTemp4_C/1
  Output Conversion Subsystem/124(Outport_124) -> GcCMS_CellTemp5_C/1
  Output Conversion Subsystem/125(Outport_125) -> GcCMS_CellTemp6_C/1
  Output Conversion Subsystem/126(Outport_126) -> GcCMS_CellTemp7_C/1
  Output Conversion Subsystem/127(Outport_127) -> GcCMS_MaxCellVoltNumb_numb/1
  Output Conversion Subsystem/128(Outport_128) -> GcCMS_MinCellVoltNumb_numb/1
  Output Conversion Subsystem/129(Outport_129) -> GcCMS_MaxCellTempNumb_numb/1
  Output Conversion Subsystem/130(Outport_130) -> GcCMS_MinCellTempNumb_numb/1
  Output Conversion Subsystem/131(Outport_131) -> GcCMS_MaxVoltNumb_numb/1
  Output Conversion Subsystem/132(Outport_132) -> GcCMS_MinVoltNumb_numb/1
  Output Conversion Subsystem/133(Outport_133) -> GcCMS_MaxTempNumb_numb/1
  Output Conversion Subsystem/134(Outport_134) -> GcCMS_MinTempNumb_numb/1
  Output Conversion Subsystem/135(Outport_135) -> GeCMS_ChgMode_enum/1
  Output Conversion Subsystem/136(Outport_136) -> GeCMS_DChrgModeDebug_enum/1
  Output Conversion Subsystem/137(Outport_137) -> GbCMS_DChrgWkUp_flg/1
  Output Conversion Subsystem/138(Outport_138) -> GeCMS_EvccMode_enum/1
  Output Conversion Subsystem/139(Outport_139) -> GeCMS_AChrgObsr_enum/1
  Output Conversion Subsystem/140(Outport_140) -> GeCMS_PreThmObsvr_enum/1
  Output Conversion Subsystem/141(Outport_141) -> GbCMS_StartCanSend_flg/1
  Output Conversion Subsystem/142(Outport_142) -> GeCMS_AppChgMode_enum/1
  Input Conversion Subsystem/1(Outport_1) -> CMS/1
  Input Conversion Subsystem/2(Outport_2) -> CMS/2
  Input Conversion Subsystem/3(Outport_3) -> CMS/3
  Input Conversion Subsystem/4(Outport_4) -> CMS/4
  Input Conversion Subsystem/5(Outport_5) -> CMS/5
  Input Conversion Subsystem/6(Outport_6) -> CMS/6
  Input Conversion Subsystem/7(Outport_7) -> CMS/7
  Input Conversion Subsystem/8(Outport_8) -> CMS/8
  Input Conversion Subsystem/9(Outport_9) -> CMS/9
  Input Conversion Subsystem/10(Outport_10) -> CMS/10
  Input Conversion Subsystem/11(Outport_11) -> CMS/11
  Input Conversion Subsystem/12(Outport_12) -> CMS/12
  Input Conversion Subsystem/13(Outport_13) -> CMS/13
  Input Conversion Subsystem/14(Outport_14) -> CMS/14
  Input Conversion Subsystem/15(Outport_15) -> CMS/15
  Input Conversion Subsystem/16(Outport_16) -> CMS/16
  Input Conversion Subsystem/17(Outport_17) -> CMS/17
  Input Conversion Subsystem/18(Outport_18) -> CMS/18
  Input Conversion Subsystem/19(Outport_19) -> CMS/19
  Input Conversion Subsystem/20(Outport_20) -> CMS/20
  Input Conversion Subsystem/21(Outport_21) -> CMS/21
  Input Conversion Subsystem/22(Outport_22) -> CMS/22
  Input Conversion Subsystem/23(Outport_23) -> CMS/23
  Input Conversion Subsystem/24(Outport_24) -> CMS/24
  Input Conversion Subsystem/25(Outport_25) -> CMS/25
  Input Conversion Subsystem/26(Outport_26) -> CMS/26
  Input Conversion Subsystem/27(Outport_27) -> CMS/27
  Input Conversion Subsystem/28(Outport_28) -> CMS/28
  Input Conversion Subsystem/29(Outport_29) -> CMS/29
  Input Conversion Subsystem/30(Outport_30) -> CMS/30
  Input Conversion Subsystem/31(Outport_31) -> CMS/31
  Input Conversion Subsystem/32(Outport_32) -> CMS/32
  Input Conversion Subsystem/33(Outport_33) -> CMS/33
  Input Conversion Subsystem/34(Outport_34) -> CMS/34
  Input Conversion Subsystem/35(Outport_35) -> CMS/35
  Input Conversion Subsystem/36(Outport_36) -> CMS/36
  Input Conversion Subsystem/37(Outport_37) -> CMS/37
  Input Conversion Subsystem/38(Outport_38) -> CMS/38
  Input Conversion Subsystem/39(Outport_39) -> CMS/39
  Input Conversion Subsystem/40(Outport_40) -> CMS/40
  Input Conversion Subsystem/41(Outport_41) -> CMS/41
  Input Conversion Subsystem/42(Outport_42) -> CMS/42
  Input Conversion Subsystem/43(Outport_43) -> CMS/43
  Input Conversion Subsystem/44(Outport_44) -> CMS/44
  Input Conversion Subsystem/45(Outport_45) -> CMS/45
  Input Conversion Subsystem/46(Outport_46) -> CMS/46
  Input Conversion Subsystem/47(Outport_47) -> CMS/47
  Input Conversion Subsystem/48(Outport_48) -> CMS/48
  Input Conversion Subsystem/49(Outport_49) -> CMS/49
  Input Conversion Subsystem/50(Outport_50) -> CMS/50
  Input Conversion Subsystem/51(Outport_51) -> CMS/51
  Input Conversion Subsystem/52(Outport_52) -> CMS/52
  Input Conversion Subsystem/53(Outport_53) -> CMS/53
  Input Conversion Subsystem/54(Outport_54) -> CMS/54
  Input Conversion Subsystem/55(Outport_55) -> CMS/55
  Input Conversion Subsystem/56(Outport_56) -> CMS/56
  Input Conversion Subsystem/57(Outport_57) -> CMS/57
  Input Conversion Subsystem/58(Outport_58) -> CMS/58
  Input Conversion Subsystem/59(Outport_59) -> CMS/59
  Input Conversion Subsystem/60(Outport_60) -> CMS/60
  Input Conversion Subsystem/61(Outport_61) -> CMS/61
  Input Conversion Subsystem/62(Outport_62) -> CMS/62
  Input Conversion Subsystem/63(Outport_63) -> CMS/63
  Input Conversion Subsystem/64(Outport_64) -> CMS/64
  Input Conversion Subsystem/65(Outport_65) -> CMS/65
  Input Conversion Subsystem/66(Outport_66) -> CMS/66
  Input Conversion Subsystem/67(Outport_67) -> CMS/67
  Input Conversion Subsystem/68(Outport_68) -> CMS/68
  Input Conversion Subsystem/69(Outport_69) -> CMS/69
  Input Conversion Subsystem/70(Outport_70) -> CMS/70
  Input Conversion Subsystem/71(Outport_71) -> CMS/71
  Input Conversion Subsystem/72(Outport_72) -> CMS/72
  Input Conversion Subsystem/73(Outport_73) -> CMS/73
  Input Conversion Subsystem/74(Outport_74) -> CMS/74
  Input Conversion Subsystem/75(Outport_75) -> CMS/75
  Input Conversion Subsystem/76(Outport_76) -> CMS/76
  Input Conversion Subsystem/77(Outport_77) -> CMS/77
  Input Conversion Subsystem/78(Outport_78) -> CMS/78
  Input Conversion Subsystem/79(Outport_79) -> CMS/79
  Input Conversion Subsystem/80(Outport_80) -> CMS/80
  Input Conversion Subsystem/81(Outport_81) -> CMS/81
  Input Conversion Subsystem/82(Outport_82) -> CMS/82
  Input Conversion Subsystem/83(Outport_83) -> CMS/83
  Input Conversion Subsystem/84(Outport_84) -> CMS/84
  Input Conversion Subsystem/85(Outport_85) -> CMS/85
  Input Conversion Subsystem/86(Outport_86) -> CMS/86
  Input Conversion Subsystem/87(Outport_87) -> CMS/87
  Input Conversion Subsystem/88(Outport_88) -> CMS/88
  Input Conversion Subsystem/89(Outport_89) -> CMS/89
  Input Conversion Subsystem/90(Outport_90) -> CMS/90
  Input Conversion Subsystem/91(Outport_91) -> CMS/91
  Input Conversion Subsystem/92(Outport_92) -> CMS/92
  Input Conversion Subsystem/93(Outport_93) -> CMS/93
  Input Conversion Subsystem/94(Outport_94) -> CMS/94
  Input Conversion Subsystem/95(Outport_95) -> CMS/95
  Input Conversion Subsystem/96(Outport_96) -> CMS/96
  Input Conversion Subsystem/97(Outport_97) -> CMS/97
  Input Conversion Subsystem/98(Outport_98) -> CMS/98
  CMS/1 -> Output Conversion Subsystem/1(Inport_1)
  CMS/2 -> Output Conversion Subsystem/2(Inport_2)
  CMS/3 -> Output Conversion Subsystem/3(Inport_3)
  CMS/4 -> Output Conversion Subsystem/4(Inport_4)
  CMS/5 -> Output Conversion Subsystem/5(Inport_5)
  CMS/6 -> Output Conversion Subsystem/6(Inport_6)
  CMS/7 -> Output Conversion Subsystem/7(Inport_7)
  CMS/8 -> Output Conversion Subsystem/8(Inport_8)
  CMS/9 -> Output Conversion Subsystem/9(Inport_9)
  CMS/10 -> Output Conversion Subsystem/10(Inport_10)
  CMS/11 -> Output Conversion Subsystem/11(Inport_11)
  CMS/12 -> Output Conversion Subsystem/12(Inport_12)
  CMS/13 -> Output Conversion Subsystem/13(Inport_13)
  CMS/14 -> Output Conversion Subsystem/14(Inport_14)
  CMS/15 -> Output Conversion Subsystem/15(Inport_15)
  CMS/16 -> Output Conversion Subsystem/16(Inport_16)
  CMS/17 -> Output Conversion Subsystem/17(Inport_17)
  CMS/18 -> Output Conversion Subsystem/18(Inport_18)
  CMS/19 -> Output Conversion Subsystem/19(Inport_19)
  CMS/20 -> Output Conversion Subsystem/20(Inport_20)
  CMS/21 -> Output Conversion Subsystem/21(Inport_21)
  CMS/22 -> Output Conversion Subsystem/22(Inport_22)
  CMS/23 -> Output Conversion Subsystem/23(Inport_23)
  CMS/24 -> Output Conversion Subsystem/24(Inport_24)
  CMS/25 -> Output Conversion Subsystem/25(Inport_25)
  CMS/26 -> Output Conversion Subsystem/26(Inport_26)
  CMS/27 -> Output Conversion Subsystem/27(Inport_27)
  CMS/28 -> Output Conversion Subsystem/28(Inport_28)
  CMS/29 -> Output Conversion Subsystem/29(Inport_29)
  CMS/30 -> Output Conversion Subsystem/30(Inport_30)
  CMS/31 -> Output Conversion Subsystem/31(Inport_31)
  CMS/32 -> Output Conversion Subsystem/32(Inport_32)
  CMS/33 -> Output Conversion Subsystem/33(Inport_33)
  CMS/34 -> Output Conversion Subsystem/34(Inport_34)
  CMS/35 -> Output Conversion Subsystem/35(Inport_35)
  CMS/36 -> Output Conversion Subsystem/36(Inport_36)
  CMS/37 -> Output Conversion Subsystem/37(Inport_37)
  CMS/38 -> Output Conversion Subsystem/38(Inport_38)
  CMS/39 -> Output Conversion Subsystem/39(Inport_39)
  CMS/40 -> Output Conversion Subsystem/40(Inport_40)
  CMS/41 -> Output Conversion Subsystem/41(Inport_41)
  CMS/42 -> Output Conversion Subsystem/42(Inport_42)
  CMS/43 -> Output Conversion Subsystem/43(Inport_43)
  CMS/44 -> Output Conversion Subsystem/44(Inport_44)
  CMS/45 -> Output Conversion Subsystem/45(Inport_45)
  CMS/46 -> Output Conversion Subsystem/46(Inport_46)
  CMS/47 -> Output Conversion Subsystem/47(Inport_47)
  CMS/48 -> Output Conversion Subsystem/48(Inport_48)
  CMS/49 -> Output Conversion Subsystem/49(Inport_49)
  CMS/50 -> Output Conversion Subsystem/50(Inport_50)
  CMS/51 -> Output Conversion Subsystem/51(Inport_51)
  CMS/52 -> Output Conversion Subsystem/52(Inport_52)
  CMS/53 -> Output Conversion Subsystem/53(Inport_53)
  CMS/54 -> Output Conversion Subsystem/54(Inport_54)
  CMS/55 -> Output Conversion Subsystem/55(Inport_55)
  CMS/56 -> Output Conversion Subsystem/56(Inport_56)
  CMS/57 -> Output Conversion Subsystem/57(Inport_57)
  CMS/58 -> Output Conversion Subsystem/58(Inport_58)
  CMS/59 -> Output Conversion Subsystem/59(Inport_59)
  CMS/60 -> Output Conversion Subsystem/60(Inport_60)
  CMS/61 -> Output Conversion Subsystem/61(Inport_61)
  CMS/62 -> Output Conversion Subsystem/62(Inport_62)
  CMS/63 -> Output Conversion Subsystem/63(Inport_63)
  CMS/64 -> Output Conversion Subsystem/64(Inport_64)
  CMS/65 -> Output Conversion Subsystem/65(Inport_65)
  CMS/66 -> Output Conversion Subsystem/66(Inport_66)
  CMS/67 -> Output Conversion Subsystem/67(Inport_67)
  CMS/68 -> Output Conversion Subsystem/68(Inport_68)
  CMS/69 -> Output Conversion Subsystem/69(Inport_69)
  CMS/70 -> Output Conversion Subsystem/70(Inport_70)
  CMS/71 -> Output Conversion Subsystem/71(Inport_71)
  CMS/72 -> Output Conversion Subsystem/72(Inport_72)
  CMS/73 -> Output Conversion Subsystem/73(Inport_73)
  CMS/74 -> Output Conversion Subsystem/74(Inport_74)
  CMS/75 -> Output Conversion Subsystem/75(Inport_75)
  CMS/76 -> Output Conversion Subsystem/76(Inport_76)
  CMS/77 -> Output Conversion Subsystem/77(Inport_77)
  CMS/78 -> Output Conversion Subsystem/78(Inport_78)
  CMS/79 -> Output Conversion Subsystem/79(Inport_79)
  CMS/80 -> Output Conversion Subsystem/80(Inport_80)
  CMS/81 -> Output Conversion Subsystem/81(Inport_81)
  CMS/82 -> Output Conversion Subsystem/82(Inport_82)
  CMS/83 -> Output Conversion Subsystem/83(Inport_83)
  CMS/84 -> Output Conversion Subsystem/84(Inport_84)
  CMS/85 -> Output Conversion Subsystem/85(Inport_85)
  CMS/86 -> Output Conversion Subsystem/86(Inport_86)
  CMS/87 -> Output Conversion Subsystem/87(Inport_87)
  CMS/88 -> Output Conversion Subsystem/88(Inport_88)
  CMS/89 -> Output Conversion Subsystem/89(Inport_89)
  CMS/90 -> Output Conversion Subsystem/90(Inport_90)
  CMS/91 -> Output Conversion Subsystem/91(Inport_91)
  CMS/92 -> Output Conversion Subsystem/92(Inport_92)
  CMS/93 -> Output Conversion Subsystem/93(Inport_93)
  CMS/94 -> Output Conversion Subsystem/94(Inport_94)
  CMS/95 -> Output Conversion Subsystem/95(Inport_95)
  CMS/96 -> Output Conversion Subsystem/96(Inport_96)
  CMS/97 -> Output Conversion Subsystem/97(Inport_97)
  CMS/98 -> Output Conversion Subsystem/98(Inport_98)
  CMS/99 -> Output Conversion Subsystem/99(Inport_99)
  CMS/100 -> Output Conversion Subsystem/100(Inport_100)
  CMS/101 -> Output Conversion Subsystem/101(Inport_101)
  CMS/102 -> Output Conversion Subsystem/102(Inport_102)
  CMS/103 -> Output Conversion Subsystem/103(Inport_103)
  CMS/104 -> Output Conversion Subsystem/104(Inport_104)
  CMS/105 -> Output Conversion Subsystem/105(Inport_105)
  CMS/106 -> Output Conversion Subsystem/106(Inport_106)
  CMS/107 -> Output Conversion Subsystem/107(Inport_107)
  CMS/108 -> Output Conversion Subsystem/108(Inport_108)
  CMS/109 -> Output Conversion Subsystem/109(Inport_109)
  CMS/110 -> Output Conversion Subsystem/110(Inport_110)
  CMS/111 -> Output Conversion Subsystem/111(Inport_111)
  CMS/112 -> Output Conversion Subsystem/112(Inport_112)
  CMS/113 -> Output Conversion Subsystem/113(Inport_113)
  CMS/114 -> Output Conversion Subsystem/114(Inport_114)
  CMS/115 -> Output Conversion Subsystem/115(Inport_115)
  CMS/116 -> Output Conversion Subsystem/116(Inport_116)
  CMS/117 -> Output Conversion Subsystem/117(Inport_117)
  CMS/118 -> Output Conversion Subsystem/118(Inport_118)
  CMS/119 -> Output Conversion Subsystem/119(Inport_119)
  CMS/120 -> Output Conversion Subsystem/120(Inport_120)
  CMS/121 -> Output Conversion Subsystem/121(Inport_121)
  CMS/122 -> Output Conversion Subsystem/122(Inport_122)
  CMS/123 -> Output Conversion Subsystem/123(Inport_123)
  CMS/124 -> Output Conversion Subsystem/124(Inport_124)
  CMS/125 -> Output Conversion Subsystem/125(Inport_125)
  CMS/126 -> Output Conversion Subsystem/126(Inport_126)
  CMS/127 -> Output Conversion Subsystem/127(Inport_127)
  CMS/128 -> Output Conversion Subsystem/128(Inport_128)
  CMS/129 -> Output Conversion Subsystem/129(Inport_129)
  CMS/130 -> Output Conversion Subsystem/130(Inport_130)
  CMS/131 -> Output Conversion Subsystem/131(Inport_131)
  CMS/132 -> Output Conversion Subsystem/132(Inport_132)
  CMS/133 -> Output Conversion Subsystem/133(Inport_133)
  CMS/134 -> Output Conversion Subsystem/134(Inport_134)
  CMS/135 -> Output Conversion Subsystem/135(Inport_135)
  CMS/136 -> Output Conversion Subsystem/136(Inport_136)
  CMS/137 -> Output Conversion Subsystem/137(Inport_137)
  CMS/138 -> Output Conversion Subsystem/138(Inport_138)
  CMS/139 -> Output Conversion Subsystem/139(Inport_139)
  CMS/140 -> Output Conversion Subsystem/140(Inport_140)
  CMS/141 -> Output Conversion Subsystem/141(Inport_141)
  CMS/142 -> Output Conversion Subsystem/142(Inport_142)
